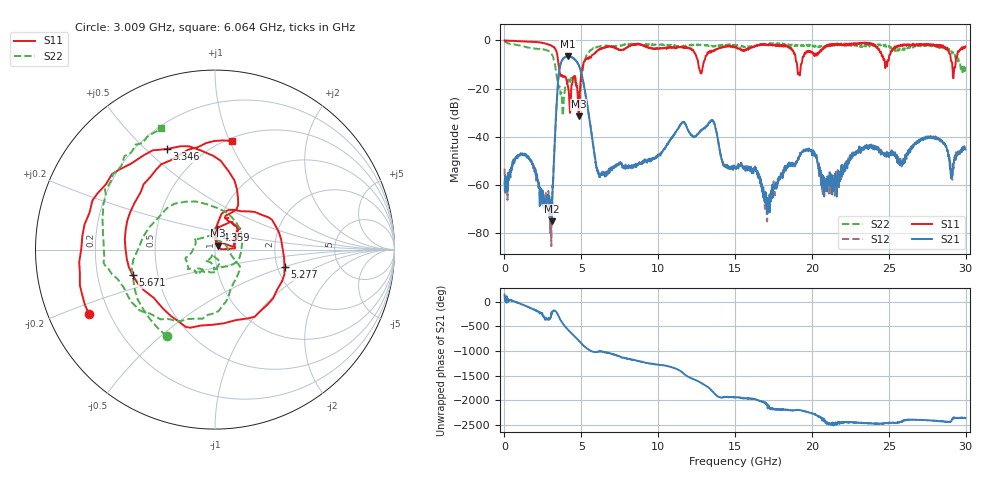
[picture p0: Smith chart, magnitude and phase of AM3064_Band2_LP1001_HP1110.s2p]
# Hz S DB R 50.0
!freq dBS11 angS11 dBS21 angS21 dBS12 angS12 dBS22 angS22
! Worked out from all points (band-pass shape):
!   1600 points, 10 MHz to 29.98 GHz, reference 50 ohm
!   highest |S21| = -6.58 dB at 4.115 GHz (marker M1); lowest = -75.0 dB at 3.065 GHz (marker M2)
!   |S21| within 3 dB of the highest: 3.665 GHz to 4.771 GHz (1.106 GHz wide, 26.2 % of centre)
!   lowest |S11| = -31.5 dB at 4.846 GHz (marker M3), VSWR 1.05, Z = 51.5 + j2.22 ohm
!   |S11| at or under -10 dB: 3.514 GHz to 5.119 GHz (1.605 GHz wide, 37.2 % of centre); 12.62 GHz to 12.93 GHz (309.8 MHz wide, 2.43 % of centre); 19.03 GHz to 19.29 GHz (260.9 MHz wide, 1.36 % of centre)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
!   |S22| runs from -31.2 to -0.3 dB; largest |S21 - S12| = 0.014
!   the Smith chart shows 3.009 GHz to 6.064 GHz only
!   S11 on the Smith chart (normalised r, x): 3.009 GHz: 0.12, -0.24; 3.346 GHz: 0.32, +0.58; 4.359 GHz: 0.99, +0.23; 5.277 GHz: 2.19, -0.50; 5.671 GHz: 0.36, -0.13; 6.064 GHz: 0.53, +1.02
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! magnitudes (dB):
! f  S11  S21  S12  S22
! 10 MHz  0.0  -58.8  -53.2  -0.3
! 1.285 GHz  -0.5  -47.7  -47.3  -2.5
! 3.009 GHz  -2.1  -71.0  -76.8  -5.2
! 3.065 GHz  -2.2  -75.0  -73.2  -5.7
! 3.346 GHz  -4.1  -32.1  -32.3  -12.8
! 3.628 GHz  -14.1  -10.4  -10.2  -21.4
! 4.115 GHz  -18.7  -6.6  -6.5  -17.2
! 4.359 GHz  -18.9  -7.0  -7.0  -15.6
! 4.846 GHz  -31.5  -10.5  -10.4  -25.2
! 5.015 GHz  -13.2  -14.1  -14.0  -15.1
! 5.277 GHz  -8.0  -22.6  -22.6  -7.1
! 5.671 GHz  -6.4  -39.2  -39.0  -3.9
! 6.064 GHz  -4.3  -54.5  -54.1  -2.6
! 10 GHz  -3.4  -47.4  -47.6  -1.8
! 13.49 GHz  -4.3  -33.1  -33.1  -2.3
! 15 GHz  -2.7  -53.1  -53.1  -1.8
! 16.41 GHz  -2.1  -54.3  -54.3  -2.1
! 17.09 GHz  -1.8  -66.4  -75.1  -1.6
! 19.99 GHz  -4.8  -45.9  -45.8  -1.9
! 21.13 GHz  -1.7  -58.2  -57.5  -2.4
! 25 GHz  -8.1  -48.5  -47.0  -2.3
! 29.98 GHz  -2.5  -45.2  -45.0  -10.9
